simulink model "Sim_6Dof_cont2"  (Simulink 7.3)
settings: Solver=ode45  StartTime=0.0  StopTime=80  FixedStep=0.0005  MaxStep=0.0002  RelTol=1e-3
StopFcn:
  | Pl
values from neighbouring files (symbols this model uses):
  calfa = cos(alfa0*d2r)    [run.m]
  d2r = pi/180    (= 0.0174532925199)    [run.m]
  klr = [0.82083770557  -0.70145835124   0.75722294555   0.32691190448   0.14993771995;        0.55253708187   0.66141640307  -0.4963339086    0.20601876795  -0.07844376733]    [run.m]
  kls = [0.23009875115  -1.3857134134    0.5565800989    0.03843893525  0.1360972015;        0.22658853965   0.3268097242   -0.0904376422    0.0272194403  -0.00768778705]    [run.m]
  r2d = 180/pi    (= 57.2957795131)    [Pl.m]    (also in run.m)
  salfa = sin(alfa0*d2r)    [run.m]
  Thet0 = 43    [run.m]
  V0 = 18640    [run.m]
undefined symbols (not defined in the file or in its folder): A6d, B6d, C6d, D6d, KJmix, KSmix

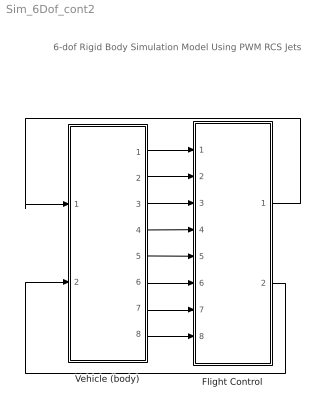
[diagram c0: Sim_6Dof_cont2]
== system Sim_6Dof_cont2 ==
  note: 6-dof Rigid Body Simulation Model Using PWM RCS Jets
  Flight Control : Subsystem
  Vehicle (body) : Subsystem
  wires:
  Vehicle (body)/2(p) -> Flight Control/2(pb)
  Vehicle (body)/3(r) -> Flight Control/3(rb)
  Vehicle (body)/6(q) -> Flight Control/6(q)
  Vehicle (body)/5(thet) -> Flight Control/5(thet)
  Vehicle (body)/7(alf) -> Flight Control/7(alfa)
  Vehicle (body)/4(bet) -> Flight Control/4(beta)
  Vehicle (body)/1(phi) -> Flight Control/1(phi)
  Flight Control/2(Aer_pqr) -> Vehicle (body)/2(Aer_pqr)
  Vehicle (body)/8(Nz) -> Flight Control/8(Nz)
  Flight Control/1(Jet_pqr) -> Vehicle (body)/1(Jet_pqr_Nz)

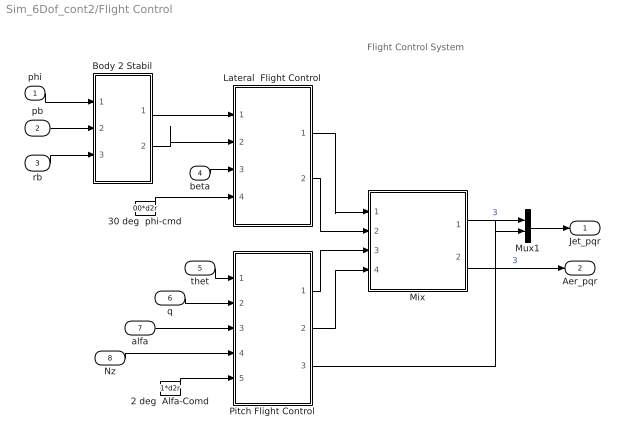
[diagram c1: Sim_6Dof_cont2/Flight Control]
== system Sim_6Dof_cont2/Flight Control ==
  note: Flight Control System
  phi : Inport  OutDataType=sfix(16)  OutScaling=2^0
  pb : Inport  Port=2  OutDataType=sfix(16)  OutScaling=2^0
  rb : Inport  Port=3  OutDataType=sfix(16)  OutScaling=2^0
  beta : Inport  Port=4  OutDataType=sfix(16)  OutScaling=2^0
  thet : Inport  Port=5  OutDataType=sfix(16)  OutScaling=2^0
  q : Inport  Port=6  OutDataType=sfix(16)  OutScaling=2^0
  alfa : Inport  Port=7  OutDataType=sfix(16)  OutScaling=2^0
  Nz : Inport  Port=8  OutDataType=sfix(16)  OutScaling=2^0
  2 deg  Alfa-Comd : Constant  Value=1*d2r  OutDataType=sfix(16)  OutScaling=2^0
  30 deg  phi-cmd : Constant  Value=00*d2r  OutDataType=sfix(16)  OutScaling=2^0
  Body 2 Stabil : Subsystem
  Lateral  Flight Control : Subsystem
  Mix : Subsystem
  Mux1 : Mux  Inputs=[3,1]
  Pitch Flight Control : Subsystem
  Jet_pqr : Outport  OutDataType=sfix(16)  OutScaling=2^0
  Aer_pqr : Outport  Port=2  OutDataType=sfix(16)  OutScaling=2^0
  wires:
  Lateral  Flight Control/1(rcs_PR) -> Mix/1(Rcs_PR)
  Lateral  Flight Control/2(aero_PR) -> Mix/2(Aer_PR)
  Pitch Flight Control/1(rcs_Q) -> Mix/3(Rcs_Q)
  Pitch Flight Control/2(aero_Q) -> Mix/4(Aer_Q)
  beta/1 -> Lateral  Flight Control/3(beta)
  Mix/2(Aer_pqr) -> Aer_pqr/1  "3"
  thet/1 -> Pitch Flight Control/1(thet)
  q/1 -> Pitch Flight Control/2(q)
  alfa/1 -> Pitch Flight Control/3(alf)
  Body 2 Stabil/2(r_s) -> Lateral  Flight Control/2(rs)
  Body 2 Stabil/1(p_s) -> Lateral  Flight Control/1(ps)
  rb/1 -> Body 2 Stabil/3(r_b)
  pb/1 -> Body 2 Stabil/2(p_b)
  phi/1 -> Body 2 Stabil/1(phi)
  Nz/1 -> Pitch Flight Control/4(Nz)
  Mix/1(Jet_pqr) -> Mux1/1  "3"
  2 deg  Alfa-Comd/1 -> Pitch Flight Control/5(alf-cmd)
  30 deg  phi-cmd/1 -> Lateral  Flight Control/4(phi-cmd)
  Pitch Flight Control/3(Nzfb) -> Mux1/2
  Mux1/1 -> Jet_pqr/1

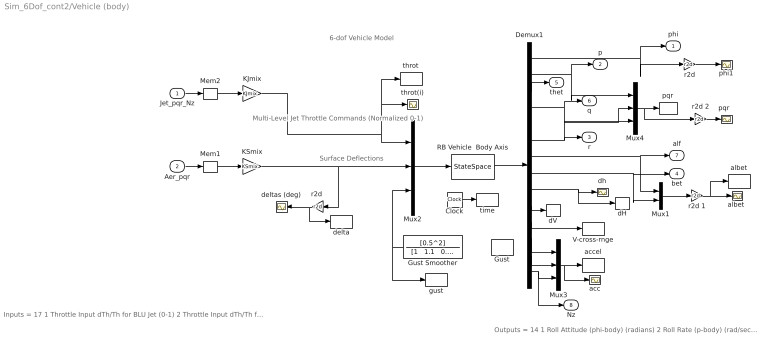
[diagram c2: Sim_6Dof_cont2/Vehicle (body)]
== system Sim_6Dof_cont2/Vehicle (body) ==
  note: Surface Deflections
  note: Multi-Level Jet Throttle Commands (Normalized 0-1)
  note: 6-dof Vehicle Model
  note: Inputs = 17 1 Throttle Input dTh/Th for BLU Jet (0-1) 2 Throttle Input dTh/Th for BRU Jet (0-1) 3 Throttle Input dTh/Th for BLD Jet (0-1) 4 Throttle Input dTh/Th for BRD Jet (0-1) 5 Throttle Input dTh/Th for BL+Y Jet (0-1) 6 Throttle Input dTh/Th for BR-Y Jet (0-1) 7 Throttle Input dTh/Th for FU Jet (0-1) 8 Throttle Input dTh/Th for FLD Jet (0-1) 9 Throttle Input dTh/Th for FRD Jet (0-1) 10 Throttle Input dTh/Th for FL+Y Jet (0-1) 11 Throttle Input dTh/Th for FR-Y Jet (0-1) 12 Left Outbrd Elevon Deflection (radians) 13 Left Inboard Elevon Deflection (radians) 14 Right Inbrd Elevon Deflection (radians) 15 Right Outbrd Elevon Deflection (radians) 16 Vertical Rudder Deflection (radians) 17 Gust Veloc, Azim-Elev Angles=(45,90) (deg)
  note: Outputs = 14 1 Roll Attitude (phi-body) (radians) 2 Roll Rate (p-body) (rad/sec) 3 Pitch Attitude (thet-bdy) (radians) 4 Pitch Rate (q-body) (rad/sec) 5 Yaw Attitude (psi-body) (radians) 6 Yaw Rate (r-body) (rad/sec) 7 Angle of attack, alfa, (radians) 8 Angle of sideslip, beta, (radian) 9 Change in Altitude, delta-h, (feet) 10 Forward Acceleration (V-dot) (ft/sec) 11 Cross Range Velocity (Vcr) (ft/sec) 12 CG Acceleration along X axis, (ft/sec^2) 13 CG Acceleration along Y axis, (ft/sec^2) 14 CG Acceleration along Z axis, (ft/sec^2)
  Jet_pqr_Nz : Inport  OutDataType=sfix(16)  OutScaling=2^0
  Aer_pqr : Inport  Port=2  OutDataType=sfix(16)  OutScaling=2^0
  Clock : Clock
  Demux1 : Demux  Outputs=14
  Gust : DiscretePulseGenerator  PulseType=Time based  Amplitude=50  Period=500  PulseWidth=10  PhaseDelay=0  SampleTime=1
  Gust Smoother : TransferFcn  Numerator=[0.5^2]  Denominator="[1   1.1   0.5^2]"
  KJmix : Gain  Gain=KJmix  Multiplication=Matrix(K*u)  ParameterDataType=sfix(16)  ParameterScaling=2^0  OutDataType=sfix(16)  OutScaling=2^0
  KSmix : Gain  Gain=KSmix  Multiplication=Matrix(K*u)  ParameterDataType=sfix(16)  ParameterScaling=2^0  OutDataType=sfix(16)  OutScaling=2^0
  Mem1 : Memory
  Mem2 : Memory
  Mux1 : Mux  Inputs=2
  Mux2 : Mux  Inputs=[11, 5, 1]
  Mux3 : Mux  Inputs=3
  Mux4 : Mux  Inputs=3
  RB Vehicle  Body Axis : StateSpace  A=A6d  B=B6d  C=C6d  D=D6d
  V-cross-rnge : ToWorkspace  VariableName=Vxrng  SampleTime=-1  SaveFormat=Array
  acc : Scope
  accel : ToWorkspace  VariableName=accel  SampleTime=-1  SaveFormat=Array
  albet : ToWorkspace  VariableName=albet  SampleTime=-1  SaveFormat=Array
  "albet " : Scope
  dH : ToWorkspace  VariableName=dH  SampleTime=-1  SaveFormat=Array
  dV : ToWorkspace  VariableName=dV  SampleTime=-1  SaveFormat=Array
  delta : ToWorkspace  VariableName=delta  SampleTime=-1  SaveFormat=Array
  deltas (deg) : Scope
  dh : Scope
  gust : ToWorkspace  VariableName=gust  SampleTime=-1  SaveFormat=Array
  phi1 : Scope
  pqr : ToWorkspace  VariableName=pqr  SampleTime=-1  SaveFormat=Array
  "pqr  " : Scope
  r2d : Gain  Gain=r2d  ParameterDataType=sfix(16)  ParameterScaling=2^0  OutDataType=sfix(16)  OutScaling=2^0
  "r2d " : Gain  Gain=r2d  ParameterDataType=sfix(16)  ParameterScaling=2^0  OutDataType=sfix(16)  OutScaling=2^0
  r2d 1 : Gain  Gain=r2d  ParameterDataType=sfix(16)  ParameterScaling=2^0  OutDataType=sfix(16)  OutScaling=2^0
  r2d 2 : Gain  Gain=r2d  ParameterDataType=sfix(16)  ParameterScaling=2^0  OutDataType=sfix(16)  OutScaling=2^0
  throt : ToWorkspace  VariableName=throt  SampleTime=-1  SaveFormat=Array
  throt(i) : Scope
  time : ToWorkspace  VariableName=time  SampleTime=-1  SaveFormat=Array
  phi : Outport  OutDataType=sfix(16)  OutScaling=2^0
  p : Outport  Port=2  OutDataType=sfix(16)  OutScaling=2^0
  r : Outport  Port=3  OutDataType=sfix(16)  OutScaling=2^0
  bet : Outport  Port=4  OutDataType=sfix(16)  OutScaling=2^0
  thet : Outport  Port=5  OutDataType=sfix(16)  OutScaling=2^0
  q : Outport  Port=6  OutDataType=sfix(16)  OutScaling=2^0
  alf : Outport  Port=7  OutDataType=sfix(16)  OutScaling=2^0
  Nz : Outport  Port=8  OutDataType=sfix(16)  OutScaling=2^0
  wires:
  Mux2/1 -> RB Vehicle  Body Axis/1
  KSmix/1 -> Mux2/2, "r2d "/1
  Demux1/2 -> p/1, Mux4/1
  Demux1/4 -> q/1, Mux4/2
  Demux1/6 -> r/1, Mux4/3
  Demux1/7 -> alf/1, Mux1/1
  Demux1/8 -> bet/1, Mux1/2
  Aer_pqr/1 -> Mem1/1
  Demux1/3 -> thet/1
  "r2d "/1 -> deltas (deg)/1, delta/1
  Demux1/1 -> phi/1, r2d/1
  RB Vehicle  Body Axis/1 -> Demux1/1
  Demux1/9 -> dh/1, dH/1
  Demux1/10 -> dV/1
  r2d 1/1 -> "albet "/1, albet/1
  Demux1/11 -> V-cross-rnge/1
  Gust Smoother/1 -> gust/1, Mux2/3
  r2d/1 -> phi1/1
  Jet_pqr_Nz/1 -> Mem2/1
  Mem1/1 -> KSmix/1
  Clock/1 -> time/1
  Mux1/1 -> r2d 1/1
  Demux1/14 -> Mux3/3, Nz/1
  Demux1/13 -> Mux3/2
  Demux1/12 -> Mux3/1
  Mux3/1 -> accel/1, acc/1
  Mux4/1 -> pqr/1, r2d 2/1
  r2d 2/1 -> "pqr  "/1
  Mem2/1 -> KJmix/1
  KJmix/1 -> Mux2/1, throt(i)/1, throt/1

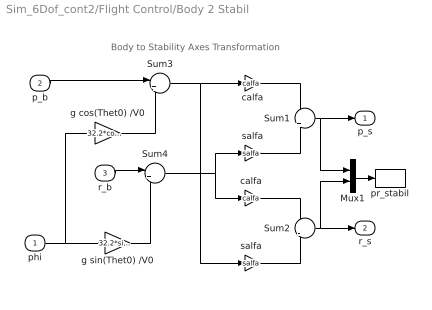
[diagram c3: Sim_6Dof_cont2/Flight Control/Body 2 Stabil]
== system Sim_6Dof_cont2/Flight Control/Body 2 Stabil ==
  note: Body to Stability Axes Transformation
  phi : Inport  OutDataType=sfix(16)  OutScaling=2^0
  p_b : Inport  Port=2  OutDataType=sfix(16)  OutScaling=2^0
  r_b : Inport  Port=3  OutDataType=sfix(16)  OutScaling=2^0
  Mux1 : Mux  Inputs=2
  Sum1 : Sum  Inputs=+|+  OutDataType=sfix(16)  OutScaling=2^0
  Sum2 : Sum  Inputs=+|-  OutDataType=sfix(16)  OutScaling=2^0
  Sum3 : Sum  Inputs=|++  OutDataType=sfix(16)  OutScaling=2^0
  Sum4 : Sum  Inputs=|+-  OutDataType=sfix(16)  OutScaling=2^0
  calfa : Gain  Gain=calfa  ParameterDataType=sfix(16)  ParameterScaling=2^0  OutDataType=sfix(16)  OutScaling=2^0
  "calfa " : Gain  Gain=calfa  ParameterDataType=sfix(16)  ParameterScaling=2^0  OutDataType=sfix(16)  OutScaling=2^0
  g cos(Thet0) /V0 : Gain  Gain=32.2*cos(Thet0*d2r)/V0  ParameterDataType=sfix(16)  ParameterScaling=2^0  OutDataType=sfix(16)  OutScaling=2^0
  g sin(Thet0) /V0 : Gain  Gain=32.2*sin(Thet0*d2r)/V0  ParameterDataType=sfix(16)  ParameterScaling=2^0  OutDataType=sfix(16)  OutScaling=2^0
  pr_stabil : ToWorkspace  VariableName=pr_st  SampleTime=-1  SaveFormat=Array
  salfa : Gain  Gain=salfa  ParameterDataType=sfix(16)  ParameterScaling=2^0  OutDataType=sfix(16)  OutScaling=2^0
  "salfa " : Gain  Gain=salfa  ParameterDataType=sfix(16)  ParameterScaling=2^0  OutDataType=sfix(16)  OutScaling=2^0
  p_s : Outport  OutDataType=sfix(16)  OutScaling=2^0
  r_s : Outport  Port=2  OutDataType=sfix(16)  OutScaling=2^0
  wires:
  Sum1/1 -> p_s/1, Mux1/1
  Sum2/1 -> r_s/1, Mux1/2
  p_b/1 -> Sum3/1
  r_b/1 -> Sum4/1
  g cos(Thet0) /V0/1 -> Sum3/2
  g sin(Thet0) /V0/1 -> Sum4/2
  phi/1 -> g cos(Thet0) /V0/1, g sin(Thet0) /V0/1
  Sum4/1 -> "calfa "/1, salfa/1
  Sum3/1 -> "salfa "/1, calfa/1
  calfa/1 -> Sum1/1
  salfa/1 -> Sum1/2
  "calfa "/1 -> Sum2/1
  "salfa "/1 -> Sum2/2
  Mux1/1 -> pr_stabil/1

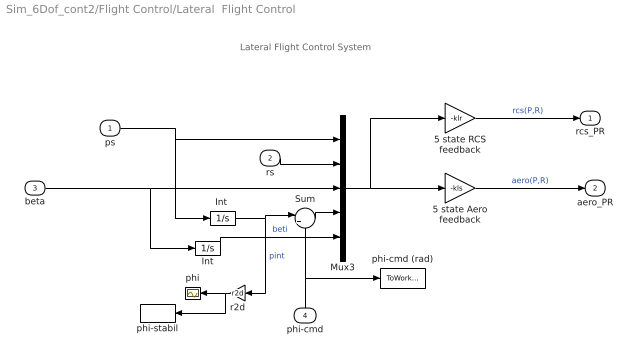
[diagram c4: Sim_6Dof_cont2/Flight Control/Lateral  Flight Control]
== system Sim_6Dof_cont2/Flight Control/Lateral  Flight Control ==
  note: Lateral Flight Control System
  ps : Inport  OutDataType=sfix(16)  OutScaling=2^0
  rs : Inport  Port=2  OutDataType=sfix(16)  OutScaling=2^0
  beta : Inport  Port=3  OutDataType=sfix(16)  OutScaling=2^0
  phi-cmd : Inport  Port=4  OutDataType=sfix(16)  OutScaling=2^0
  5 state Aero feedback : Gain  Gain=-kls  Multiplication=Matrix(K*u)  ParameterDataType=sfix(16)  ParameterScaling=2^0  OutDataType=sfix(16)  OutScaling=2^0
  5 state RCS feedback : Gain  Gain=-klr  Multiplication=Matrix(K*u)  ParameterDataType=sfix(16)  ParameterScaling=2^0  OutDataType=sfix(16)  OutScaling=2^0
  Int : Integrator
  "Int " : Integrator
  Mux3 : Mux  Inputs=5
  Sum : Sum  Inputs=|+-  OutDataType=sfix(16)  OutScaling=2^0
  phi : Scope
  phi-cmd (rad) : ToWorkspace  VariableName=phi_cmd  SampleTime=-1  SaveFormat=Array
  phi-stabil : ToWorkspace  VariableName=phi_st  SampleTime=-1  SaveFormat=Array
  r2d : Gain  Gain=r2d  ParameterDataType=sfix(16)  ParameterScaling=2^0  OutDataType=sfix(16)  OutScaling=2^0
  rcs_PR : Outport  OutDataType=sfix(16)  OutScaling=2^0
  aero_PR : Outport  Port=2  OutDataType=sfix(16)  OutScaling=2^0
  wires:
  "Int "/1 -> Sum/1, r2d/1  "pint"
  Sum/1 -> Mux3/4
  Int/1 -> Mux3/5  "beti"
  beta/1 -> Int/1, Mux3/3
  ps/1 -> "Int "/1, Mux3/1
  Mux3/1 -> 5 state Aero feedback/1, 5 state RCS feedback/1
  rs/1 -> Mux3/2
  5 state RCS feedback/1 -> rcs_PR/1  "rcs(P,R)"
  5 state Aero feedback/1 -> aero_PR/1  "aero(P,R)"
  phi-cmd/1 -> Sum/2, phi-cmd (rad)/1
  r2d/1 -> phi/1, phi-stabil/1

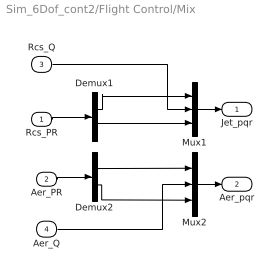
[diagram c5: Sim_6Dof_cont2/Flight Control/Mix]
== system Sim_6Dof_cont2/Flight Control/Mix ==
  Rcs_PR : Inport  OutDataType=sfix(16)  OutScaling=2^0
  Aer_PR : Inport  Port=2  OutDataType=sfix(16)  OutScaling=2^0
  Rcs_Q : Inport  Port=3  OutDataType=sfix(16)  OutScaling=2^0
  Aer_Q : Inport  Port=4  OutDataType=sfix(16)  OutScaling=2^0
  Demux1 : Demux  Outputs=2
  Demux2 : Demux  Outputs=2
  Mux1 : Mux  Inputs=3
  Mux2 : Mux  Inputs=3
  Jet_pqr : Outport  OutDataType=sfix(16)  OutScaling=2^0
  Aer_pqr : Outport  Port=2  OutDataType=sfix(16)  OutScaling=2^0
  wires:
  Demux1/1 -> Mux1/1
  Demux1/2 -> Mux1/3
  Demux2/1 -> Mux2/1
  Demux2/2 -> Mux2/3
  Mux1/1 -> Jet_pqr/1
  Rcs_PR/1 -> Demux1/1
  Aer_PR/1 -> Demux2/1
  Aer_Q/1 -> Mux2/2
  Mux2/1 -> Aer_pqr/1
  Rcs_Q/1 -> Mux1/2

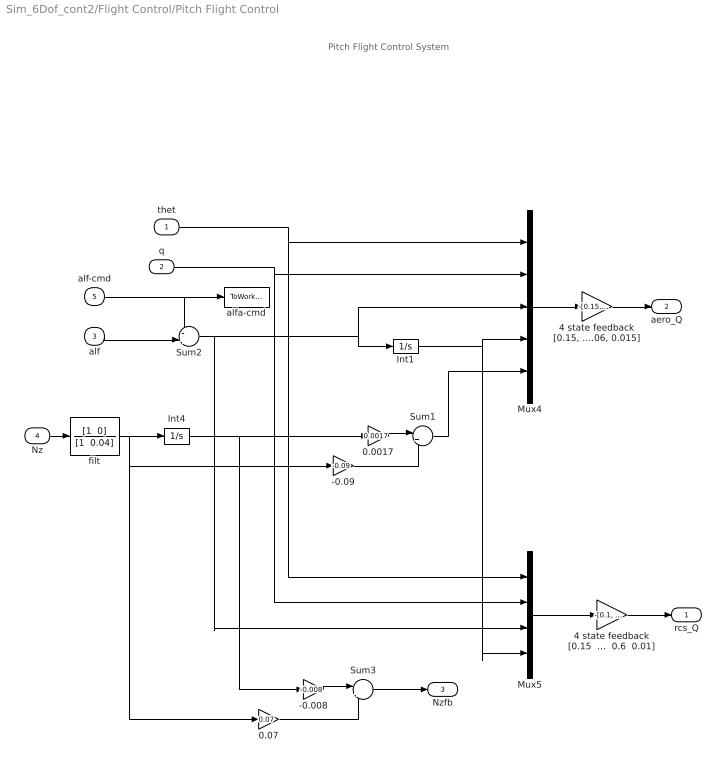
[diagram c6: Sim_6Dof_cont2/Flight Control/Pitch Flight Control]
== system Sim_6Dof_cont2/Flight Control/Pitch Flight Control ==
  note: Pitch Flight Control System
  thet : Inport  OutDataType=sfix(16)  OutScaling=2^0
  q : Inport  Port=2  OutDataType=sfix(16)  OutScaling=2^0
  alf : Inport  Port=3  OutDataType=sfix(16)  OutScaling=2^0
  Nz : Inport  Port=4  OutDataType=sfix(16)  OutScaling=2^0
  alf-cmd : Inport  Port=5  OutDataType=sfix(16)  OutScaling=2^0
  -0.008 : Gain  Gain=-0.008  ParameterDataType=sfix(16)  ParameterScaling=2^0  OutDataType=sfix(16)  OutScaling=2^0
  -0.09 : Gain  Gain=-0.09  ParameterDataType=sfix(16)  ParameterScaling=2^0  OutDataType=sfix(16)  OutScaling=2^0
  0.0017 : Gain  Gain=0.0017  ParameterDataType=sfix(16)  ParameterScaling=2^0  OutDataType=sfix(16)  OutScaling=2^0
  0.07 : Gain  Gain=0.07  ParameterDataType=sfix(16)  ParameterScaling=2^0  OutDataType=sfix(16)  OutScaling=2^0
  4 state feedback [0.15  1.8  0.6  0.01] : Gain  Gain="-[0.1,   1.8,   0.8,    0.01]"  Multiplication=Matrix(K*u)  ParameterDataType=sfix(16)  ParameterScaling=2^0  OutDataType=sfix(16)  OutScaling=2^0
  "4 state feedback [0.15, 2, 0.9, 0.06, 0.015]" : Gain  Gain="-[0.15,   2,   0.9,    0.08,   0.015]"  Multiplication=Matrix(K*u)  ParameterDataType=sfix(16)  ParameterScaling=2^0  OutDataType=sfix(16)  OutScaling=2^0
  Int1 : Integrator
  Int4 : Integrator
  Mux4 : Mux  Inputs=5
  Mux5 : Mux
  Sum1 : Sum  Inputs=|++  OutDataType=sfix(16)  OutScaling=2^0
  Sum2 : Sum  Inputs=-+|  OutDataType=sfix(16)  OutScaling=2^0
  Sum3 : Sum  Inputs=|++  OutDataType=sfix(16)  OutScaling=2^0
  alfa-cmd : ToWorkspace  VariableName=alfa_cmd  SampleTime=-1  SaveFormat=Array
  filt : TransferFcn  Numerator="[1  0]"  Denominator="[1  0.04]"
  rcs_Q : Outport  OutDataType=sfix(16)  OutScaling=2^0
  aero_Q : Outport  Port=2  OutDataType=sfix(16)  OutScaling=2^0
  Nzfb : Outport  Port=3  OutDataType=sfix(16)  OutScaling=2^0
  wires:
  alf-cmd/1 -> Sum2/1, alfa-cmd/1
  alf/1 -> Sum2/2
  filt/1 -> 0.07/1, -0.09/1, Int4/1
  Int4/1 -> -0.008/1, 0.0017/1
  -0.008/1 -> Sum3/1
  0.07/1 -> Sum3/2
  4 state feedback [0.15  1.8  0.6  0.01]/1 -> rcs_Q/1
  Mux5/1 -> 4 state feedback [0.15  1.8  0.6  0.01]/1
  "4 state feedback [0.15, 2, 0.9, 0.06, 0.015]"/1 -> aero_Q/1
  Mux4/1 -> "4 state feedback [0.15, 2, 0.9, 0.06, 0.015]"/1
  Sum1/1 -> Mux4/5
  Nz/1 -> filt/1
  -0.09/1 -> Sum1/2
  0.0017/1 -> Sum1/1
  q/1 -> Mux5/2, Mux4/2
  thet/1 -> Mux5/1, Mux4/1
  Sum2/1 -> Mux5/3, Mux4/3, Int1/1
  Int1/1 -> Mux5/4, Mux4/4
  Sum3/1 -> Nzfb/1
